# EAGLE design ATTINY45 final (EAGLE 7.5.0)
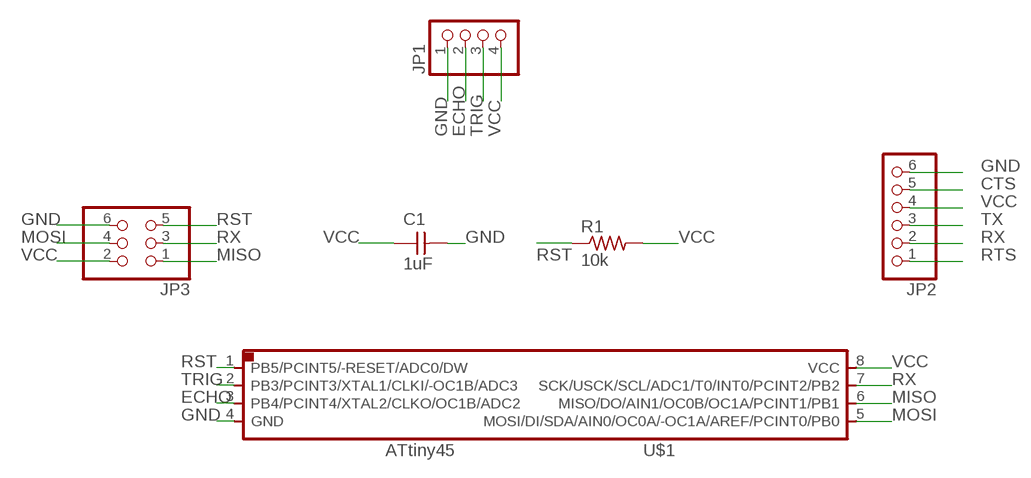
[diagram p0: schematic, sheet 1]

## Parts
C1  1uF  CAP-UNPOLARIZEDFAB  [C1206FAB]
JP1  PINHD-1X4  [1X04]
JP2  PINHD-1X6  [1X06]
JP3  PINHD-2X3  [2X03]
R1  10k  RES-US1206FAB  [R1206FAB]
U$1  ATTINY45SI  [SOIC8]

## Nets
CTS: JP2.5
ECHO: JP1.2 U$1.3(PB4/PCINT4/XTAL2/CLKO/OC1B/ADC2)
GND: C1.2 JP1.1 JP2.6 JP3.6 U$1.4(GND)
MISO: JP3.1 U$1.6(MISO/DO/AIN1/OC0B/OC1A/PCINT1/PB1)
MOSI: JP3.4 U$1.5(MOSI/DI/SDA/AIN0/OC0A/-OC1A/AREF/PCINT0/PB0)
RST: JP3.5 R1.1 U$1.1(PB5/PCINT5/-RESET/ADC0/DW)
RTS: JP2.1
RX: JP2.2 JP3.3 U$1.7(SCK/USCK/SCL/ADC1/T0/INT0/PCINT2/PB2)
TRIG: JP1.3 U$1.2(PB3/PCINT3/XTAL1/CLKI/-OC1B/ADC3)
TX: JP2.3
VCC: C1.1 JP1.4 JP2.4 JP3.2 R1.2 U$1.8(VCC)

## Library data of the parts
C1 = fab:CAP-UNPOLARIZED
JP1 = pinhead:PINHD-1X4: PIN HEADER
JP2 = pinhead:PINHD-1X6: PIN HEADER
JP3 = pinhead:PINHD-2X3: PIN HEADER
R1 = fab:RES-US: Resistor (US Symbol)
U$1 = fab:ATTINY45

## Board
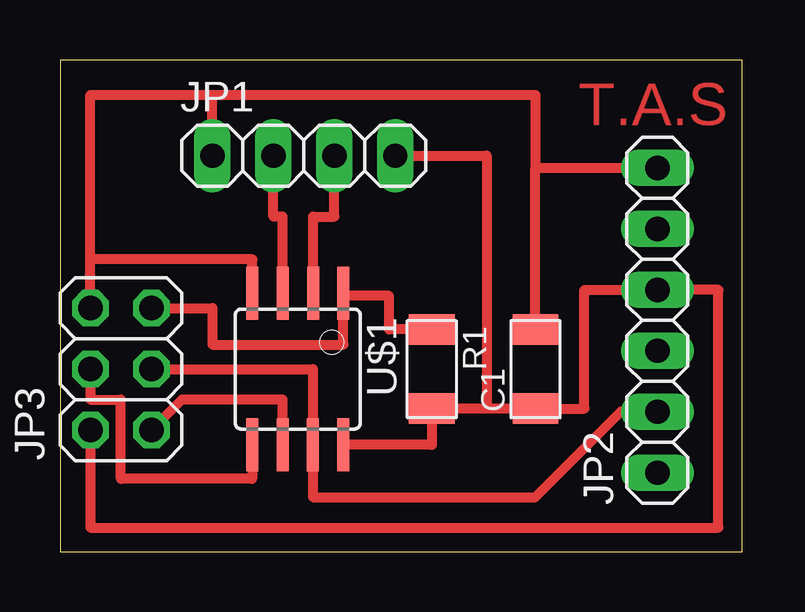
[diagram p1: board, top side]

Size 28.43 x 20.5 mm. Coordinates in mm from the lower left corner, seen from the top.
Outline: 0,0 28.43,0 28.43,20.5 0,20.5 0,0
Copper layers (1*16): Top 0.035mm / dielectric 1.5mm / Bottom 0.035mm
Design rules "default": minimum track width 10mil, minimum drill 24mil, track to track 8mil, track to pad 8mil, pad to pad 8mil, via to via 8mil, smd to smd 8mil, copper to edge 40mil, drill to drill 8mil, minimum pad ring 10mil, minimum via ring 8mil, stop-mask expansion 4mil, vias tented up to drill 0mil, thermal gap 10mil

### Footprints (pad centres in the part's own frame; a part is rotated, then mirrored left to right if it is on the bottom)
C1206FAB = smd 1.27 x 1.905: 1 -1.651,0; 2 1.651,0
1X04 = drill 1.016 long: 1 -3.81,0; 2 -1.27,0; 3 1.27,0; 4 3.81,0
1X06 = drill 1.016 long: 1 -6.35,0; 2 -3.81,0; 3 -1.27,0; 4 1.27,0; 5 3.81,0; 6 6.35,0
2X03 = drill 1.016 octagon: 1 -2.54,-1.27; 2 -2.54,1.27; 3 0,-1.27; 4 0,1.27; 5 2.54,-1.27; 6 2.54,1.27
R1206FAB = smd 1.27 x 1.905: 1 -1.651,0; 2 1.651,0
SOIC8 = smd 0.5 x 2.2: 1 -1.905,-3.154; 2 -0.645,-3.154; 3 0.625,-3.154; 4 1.895,-3.154; 5 1.905,3.154; 6 0.635,3.154; 7 -0.635,3.154; 8 -1.905,3.154

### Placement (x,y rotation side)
C1  19.81,7.62 90 top
JP1  10.16,16.51 0 top
JP2  24.89,9.65 90 top
JP3  2.54,7.62 90 top
R1  15.49,7.62 270 top
U$1  9.91,7.62 180 top

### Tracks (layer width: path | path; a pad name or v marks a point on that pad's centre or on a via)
ECHO
  Top 0.406: U$1.3 9.28,13.97 8.89,13.97 JP1.2
GND
  Top 0.406: C1.2 19.81,16 | 19.81,16 JP2.6 | JP1.1 6.35,19.05 | 6.35,19.05 19.81,19.05 19.81,16 | JP3.6 1.27,12.19 | 1.27,12.19 1.27,19.05 6.35,19.05 | U$1.4 8.01,12.19 1.27,12.19
MISO
  Top 0.406: U$1.6 9.27,6.35 5.08,6.35 JP3.1
MOSI
  Top 0.406: JP3.4 1.27,6.35 2.54,6.35 2.54,3.05 8,3.05 U$1.5
RST
  Top 0.406: 15.49,9.14 R1.1 13.72,9.27 13.72,10.67 11.81,10.67 U$1.1 11.81,8.64 6.35,8.64 6.35,10.16 JP3.5
RX
  Top 0.406: JP3.3 10.54,7.62 U$1.7 10.54,2.29 19.81,2.29 23.37,5.84 JP2.2
TRIG
  Top 0.406: U$1.2 10.55,13.97 11.43,13.97 JP1.3
VCC
  Top 0.406: U$1.8 15.49,4.47 R1.2 17.78,5.97 | 17.78,5.97 C1.1 21.84,5.97 21.84,10.92 JP2.4 27.43,10.92 27.43,1.02 1.27,1.02 JP3.2 | JP1.4 17.78,16.51 17.78,5.97

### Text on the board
Top: T.A.S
